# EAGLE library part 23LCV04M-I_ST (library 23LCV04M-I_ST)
SRAM 4Mbit serial SRAM, 2.2V-3.6V with Battery Backup Source: Datasheet
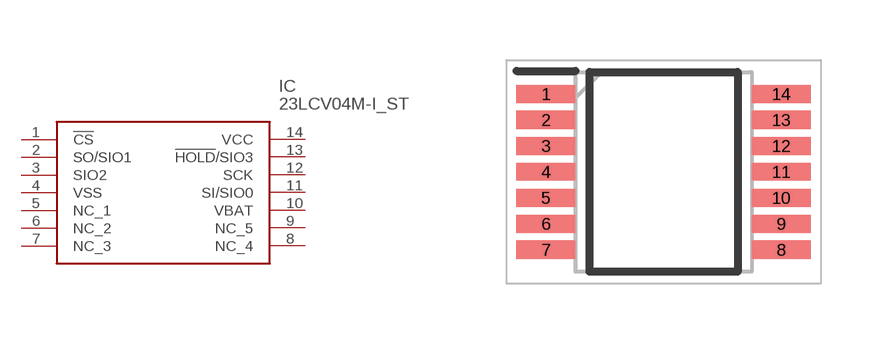
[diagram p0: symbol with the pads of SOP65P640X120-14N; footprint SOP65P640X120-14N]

Designator prefix IC

## 23LCV04M-I_ST (Description: SRAM 4Mbit serial SRAM, 2.2V-3.6V with Battery Backup; Height: 1.2mm; Manufacturer_Name: Microchip; Manufacturer_Part_Number: 23LCV04M-I/ST)  [SOP65P640X120-14N]
1  !CS
2  SO/SIO1
3  SIO2
4  VSS
5  NC_1
6  NC_2
7  NC_3
8  NC_4
9  NC_5
10  VBAT
11  SI/SIO0
12  SCK
13  !HOLD!/SIO3
14  VCC

## Footprint SOP65P640X120-14N (pad centres in mm)
**14-Lead Plastic Thin Shrink Small Outline (ST) &ndash; 4.4 mm (TSSOP)
smd 1.475 x 0.45: 1 -2.938,1.95; 2 -2.938,1.3; 3 -2.938,0.65; 4 -2.938,0; 5 -2.938,-0.65; 6 -2.938,-1.3; 7 -2.938,-1.95; 8 2.938,-1.95; 9 2.938,-1.3; 10 2.938,-0.65; 11 2.938,0; 12 2.938,0.65; 13 2.938,1.3; 14 2.938,1.95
